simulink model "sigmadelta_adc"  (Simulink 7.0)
settings: Solver=ode45  StartTime=0.0  StopTime=(kmod+nmod)/fmod  RelTol=1e-3
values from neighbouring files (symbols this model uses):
  A1 = 0    [go_sigmadelta_adc.m]
  A2 = 0    [go_sigmadelta_adc.m]
  acmag = 0.5    [go_sigmadelta_adc.m]
  F1 = 40E3    (= 40000)    [go_sigmadelta_adc.m]
  F2 = 20E3    (= 20000)    [go_sigmadelta_adc.m]
  fmod = 8E3    (= 8000)    [go_sigmadelta_adc.m]
  tQ = 1/(2*osr*fmod)    (= 9.765625e-07)    [go_sigmadelta_adc.m]
undefined symbols (not defined in the file or in its folder): fq
libraries: simulink x1

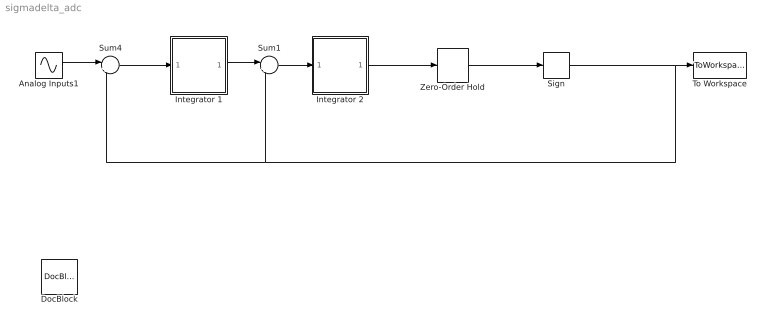
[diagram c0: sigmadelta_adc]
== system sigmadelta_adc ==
  Analog Inputs1 : Sin  Amplitude=acmag  Frequency=2*pi*fmod  Samples=round(fq/fmod)  SampleTime=tQ
  DocBlock : simulink/Model-Wide Utilities/DocBlock  SystemSampleTime=-1  DocumentType=Text
  Integrator 1 : Subsystem  mask{F=F1, A=A1, ic=0}
      mask prompts: F "Gm/C factor (integrator scaling)"; A "Integrator (max) Gain"; ic "Initial Condition"
  Integrator 2 : Subsystem  mask{F=F2, A=A2, ic=0}
      mask prompts: F "Gm/C factor (integrator scaling)"; A "Integrator (max) Gain"; ic "Initial Condition"
  Sign : Signum
  Sum1 : Sum  Inputs=|+-  OutDataType=sfix(16)  OutScaling=2^0
  Sum4 : Sum  Inputs=|+-  OutDataType=sfix(16)  OutScaling=2^0
  To Workspace : ToWorkspace  VariableName=yout  SampleTime=tQ  SaveFormat=Array
  Zero-Order Hold : ZeroOrderHold  SampleTime=tQ
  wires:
  Analog Inputs1/1 -> Sum4/1
  Zero-Order Hold/1 -> Sign/1
  Sign/1 -> To Workspace/1, Sum4/2, Sum1/2
  Integrator 2/1(Out1) -> Zero-Order Hold/1
  Sum4/1 -> Integrator 1/1(In1)
  Integrator 1/1(Out1) -> Sum1/1
  Sum1/1 -> Integrator 2/1(In1)

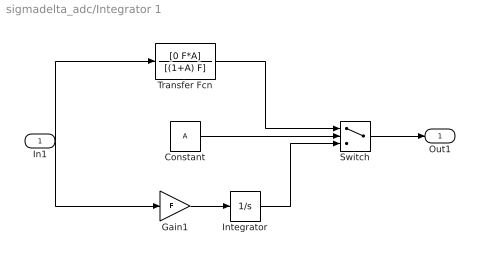
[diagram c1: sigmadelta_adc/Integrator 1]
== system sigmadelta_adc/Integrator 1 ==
  In1 : Inport  OutDataType=sfix(16)  OutScaling=2^0
  Constant : Constant  Value=A  OutDataType=sfix(16)  OutScaling=2^0
  Gain1 : Gain  Gain=F  ParameterDataType=sfix(16)  ParameterScaling=2^0  OutDataType=sfix(16)  OutScaling=2^0
  Integrator : Integrator  InitialCondition=ic
  Switch : Switch  Criteria=u2 ~= 0
  Transfer Fcn : TransferFcn  Numerator=[0 F*A]  Denominator=[(1+A) F]
  Out1 : Outport  OutDataType=sfix(16)  OutScaling=2^0
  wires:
  Transfer Fcn/1 -> Switch/1
  Constant/1 -> Switch/2
  Integrator/1 -> Switch/3
  Switch/1 -> Out1/1
  In1/1 -> Transfer Fcn/1, Gain1/1
  Gain1/1 -> Integrator/1

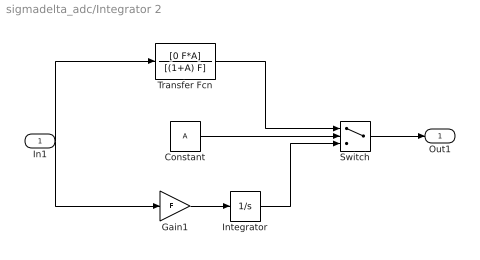
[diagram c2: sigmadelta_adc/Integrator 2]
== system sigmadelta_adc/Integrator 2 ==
  In1 : Inport  OutDataType=sfix(16)  OutScaling=2^0
  Constant : Constant  Value=A  OutDataType=sfix(16)  OutScaling=2^0
  Gain1 : Gain  Gain=F  ParameterDataType=sfix(16)  ParameterScaling=2^0  OutDataType=sfix(16)  OutScaling=2^0
  Integrator : Integrator  InitialCondition=ic
  Switch : Switch  Criteria=u2 ~= 0
  Transfer Fcn : TransferFcn  Numerator=[0 F*A]  Denominator=[(1+A) F]
  Out1 : Outport  OutDataType=sfix(16)  OutScaling=2^0
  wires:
  Gain1/1 -> Integrator/1
  In1/1 -> Gain1/1, Transfer Fcn/1
  Switch/1 -> Out1/1
  Integrator/1 -> Switch/3
  Constant/1 -> Switch/2
  Transfer Fcn/1 -> Switch/1
